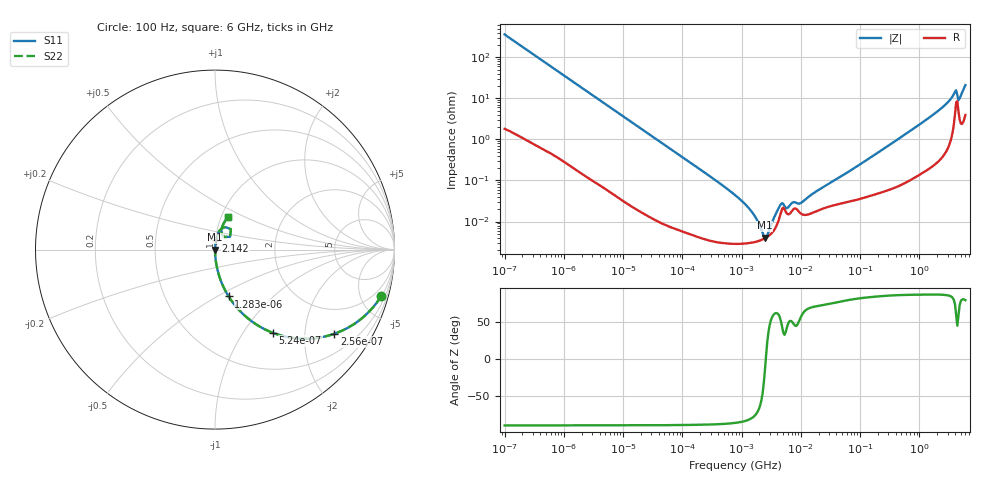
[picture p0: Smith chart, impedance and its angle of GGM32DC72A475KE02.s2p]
!Murata Part Number: GGM32DC72A475KE02
!These Parameters are Measured in Series Mode Connection
!Data Generated on Jun 19, 2026
!  o--ll--o
!Port1  Port2
!  o------o
!Operation Temp=25[degC], DC Bias Voltage=0[V]
!Freq. Start=100[Hz] Stop=6[GHz] 401[Steps]
# Hz S RI R 50
!Freq.(Hz) S11(Real) S11(Imag) S21(Real) S21(Imag) S12(Real) S12(Imag) S22(Real) S22(Imag)
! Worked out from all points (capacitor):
!   401 points, 100 Hz to 6 GHz, reference 50 ohm
!   read as one part in series: C = 4.42 uF near 109 Hz
!   lowest |Z| = 4.04 mohm at 2.481 MHz (marker M1)
!   series resonance near 2.566 MHz, so ESL is about 870 pH
!   S11 on the Smith chart (normalised r, x): 100 Hz: 1.04, -7.19; 256 Hz: 1.02, -2.82; 524 Hz: 1.01, -1.38; 1.283 kHz: 1.00, -0.57; 2.142 GHz: 1.01, +0.10; 6 GHz: 1.08, +0.41
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100  0.9271 -0.2575  0.0729 0.2575  0.0729 0.2575  0.9271 -0.2575
256  0.6641 -0.4692  0.3359 0.4692  0.3359 0.4692  0.6641 -0.4692
524  0.3241 -0.4644  0.6759 0.4644  0.6759 0.4644  0.3241 -0.4644
1283  0.0761 -0.2613  0.9239 0.2613  0.9239 0.2613  0.0761 -0.2613
2008  0.0332 -0.1752  0.9668 0.1752  0.9668 0.1752  0.0332 -0.1752
6433  0.00372 -0.0568  0.9963 0.0568  0.9963 0.0568  0.00372 -0.0568
40335  0.000181 -0.00917  0.9998 0.00917  0.9998 0.00917  0.000181 -0.00917
774597  2.88e-05 -0.000442  1 0.000442  1 0.000442  2.88e-05 -0.000442
1267578  2.97e-05 -0.000226  1 0.000226  1 0.000226  2.97e-05 -0.000226
1896632  3.33e-05 -9.23e-05  1 9.23e-05  1 9.23e-05  3.33e-05 -9.23e-05
2481164  3.91e-05 -1.03e-05  1 1.03e-05  1 1.03e-05  3.91e-05 -1.03e-05
3245845  5.28e-05 7.69e-05  0.9999 -7.69e-05  0.9999 -7.69e-05  5.28e-05 7.69e-05
4643984  0.000172 0.000206  0.9998 -0.000206  0.9998 -0.000206  0.000172 0.000206
5809218  0.000157 0.000141  0.9998 -0.000141  0.9998 -0.000141  0.000157 0.000141
7599586  0.000203 0.000217  0.9998 -0.000217  0.9998 -0.000217  0.000203 0.000217
9941735  0.000158 0.000233  0.9998 -0.000233  0.9998 -0.000233  0.000158 0.000233
1.555665e7  0.000162 0.000436  0.9998 -0.000436  0.9998 -0.000436  0.000162 0.000436
3.124326e8  0.000647 0.00728  0.9994 -0.00728  0.9994 -0.00728  0.000647 0.00728
2.142435e9  0.00557 0.0507  0.9944 -0.0507  0.9944 -0.0507  0.00557 0.0507
3.8344e9  0.0373 0.1177  0.9627 -0.1177  0.9627 -0.1177  0.0373 0.1177
4.796499e9  0.0376 0.0888  0.9624 -0.0888  0.9624 -0.0888  0.0376 0.0888
6e9  0.0746 0.184  0.9254 -0.184  0.9254 -0.184  0.0746 0.184
